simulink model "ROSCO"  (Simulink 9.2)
settings: Solver=VariableStepAuto  StartTime=0.0  StopTime=TMax  RelTol=1e-3
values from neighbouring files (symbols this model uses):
  OutList = [OutList    [runFAST.m]    (also in ROSCO2Matlab.m = [])
undefined symbols (not defined in the file or in its folder): cosd, DiscIntNeverNeededParam, F, Parameter, R, rpm2radps, simu, sind, strmatch
libraries: simulink x10
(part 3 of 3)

== matlab function Cyclic Pitch controller/1P Cyclic Pitch Controller1/saturation
(limit schedule)1 ==
%limit b_d and b_q so b_1,2,or3 does not get bigger than b_avg (the sinusoids don't get cut off at zero)
%unless b_avg is <0, then limit to 0
%at_limit is 1 if limited, 0 otherwise

function [bdq,k]  = fcn(bdq_unsat, b_avg, M0,minPitch,Params)

MODE    = Params(1);  % 1 no IPC below rated (no power loss), 2 IPC always on, 3 depends on mean load
M0_set  = Params(2);
k_sat   = Params(3);

if MODE == 1
    
    if (b_avg <= minPitch)
        bdq=[0;0];
        k = 0;
    else
        if (norm(bdq_unsat,2) <= b_avg - minPitch)
            bdq = bdq_unsat;
            k = 1;
        else
            bdq=bdq_unsat*((b_avg-minPitch)/norm(bdq_unsat,2));
            k = (b_avg/norm(bdq_unsat,2));
        end
    end
elseif MODE == 2
    if (norm(bdq_unsat,2) > deg2rad(15))
        bdq = bdq_unsat*(deg2rad(15)/norm(bdq_unsat,2));
        k = (deg2rad(15)/norm(bdq_unsat,2));
    else
        bdq = bdq_unsat;
        k = 1;
    end
else  % MODE 3
    if (M0 > M0_set - 1/(2*k_sat))
        if (M0 > M0_set + 1/(2*k_sat))
            bdq = bdq_unsat;
            k = 1;
        else
            k = k_sat*(M0-M0_set)+1/2;
            bdq = k*bdq_unsat;
        end
    else
        bdq = [0;0];
        k = 0;
    end
end
%
% if (b_avg <=0)
%         bdq = bdq_unsat;
% else
%     if (norm(bdq_unsat,2) <= b_avg)
%         bdq = bdq_unsat;
%     else
%         bdq = bdq_unsat;
%     end
% end

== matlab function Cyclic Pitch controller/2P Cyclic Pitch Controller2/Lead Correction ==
function [b_cos,b_sin] = fcn(bdq, psi_o)
% This block supports the Embedded MATLAB subset.
% See the help menu for details. 

b_cos=[cosd(psi_o) sind(psi_o)]*bdq;
b_sin=[-sind(psi_o) cosd(psi_o)]*bdq;

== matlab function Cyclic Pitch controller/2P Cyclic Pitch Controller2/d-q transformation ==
function [M_tilt,M_yaw] = fwdMBC2(RootMyb, Az, NumBl)
% This block supports the Embedded MATLAB subset.
% See the help menu for details.

if NumBl == 2
    
    My=RootMyb-mean(RootMyb(1:2)); %remove mean
    
    M_tilt = [cosd(2*Az) cosd(2*(Az+180)) 0]*My;
    M_yaw =  [sind(2*Az) sind(2*(Az+180)) 0]*My;
else
    My=RootMyb-mean(RootMyb); %remove mean
    
    M_tilt = [cosd(2*Az) cosd(2*(Az+120)) cosd(2*(Az+240))]*My;
    M_yaw =  [sind(2*Az) sind(2*(Az+120)) sind(2*(Az+240))]*My;
end

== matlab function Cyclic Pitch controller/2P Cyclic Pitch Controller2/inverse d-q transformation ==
function [b1,b2,b3] = bckMBC2(bdq, Az, NumBl)
% This block supports the Embedded MATLAB subset.
% See the help menu for details.


if NumBl == 2
    
    b1=[cosd(2*Az) sind(2*Az)]*bdq;
    b2=[cosd(2*(Az - 180)) sind(2*(Az - 180))]*bdq;
    b3=0;
    
else
    b1=[cosd(2*Az) sind(2*Az)]*bdq;
    b2=[cosd(2*(Az + 120)) sind(2*(Az + 120))]*bdq;
    b3=[cosd(2*(Az + 240)) sind(2*(Az + 240))]*bdq;
    
end

== matlab function Cyclic Pitch controller/2P Cyclic Pitch Controller2/saturation
(limit schedule)1 ==
%limit b_d and b_q so b_1,2,or3 does not get bigger than b_avg (the sinusoids don't get cut off at zero)
%unless b_avg is <0, then limit to 0
%at_limit is 1 if limited, 0 otherwise

function [bdq,k]  = fcn(bdq_unsat, b_avg, M0,minPitch,Params)

MODE    = Params(1);  % 1 no IPC below rated (no power loss), 2 IPC always on, 3
M0_set  = Params(2);
k_sat   = Params(3);

if MODE == 1
    
    if (b_avg <= minPitch)
        bdq=[0;0];
        k = 0;
    else
        if (norm(bdq_unsat,2) <= b_avg - minPitch)
            bdq = bdq_unsat;
            k = 1;
        else
            bdq=bdq_unsat*((b_avg-minPitch)/norm(bdq_unsat,2));
            k = (b_avg/norm(bdq_unsat,2));
        end
    end
elseif MODE == 2
    if (norm(bdq_unsat,2) > deg2rad(15))
        bdq = bdq_unsat*(deg2rad(15)/norm(bdq_unsat,2));
        k = (deg2rad(15)/norm(bdq_unsat,2));
    else
        bdq = bdq_unsat;
        k = 1;
    end
else  % MODE 3
    if (M0 > M0_set - 1/(2*k_sat))
        if (M0 > M0_set + 1/(2*k_sat))
            bdq = bdq_unsat;
            k = 1;
        else
            k = k_sat*(M0-M0_set)+1/2;
            bdq = k*bdq_unsat;
        end
    else
        bdq = [0;0];
        k = 0;
    end
end
%
% if (b_avg <=0)
%         bdq = bdq_unsat;
% else
%     if (norm(bdq_unsat,2) <= b_avg)
%         bdq = bdq_unsat;
%     else
%         bdq = bdq_unsat;
%     end
% end
